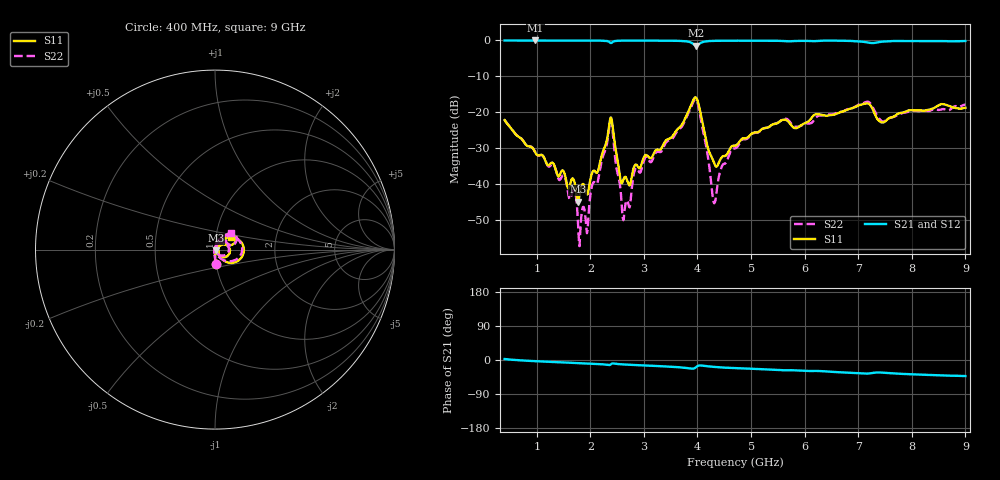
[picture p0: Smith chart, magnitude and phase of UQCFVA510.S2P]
!  Part Number  UQCFVA510  Mounting Orientation: Horizontal
!  Description: Ultra Low ESR Microwave capacitors
!  Application: Coupling, Bypass, Tuning, DC Block
!  Filters, Matching
# GHZ S DB R 50
! Freq  |S11|  S11 Ph  |S21|  S21 Ph  |S12|  S12 Ph  |S22|  S22 Ph
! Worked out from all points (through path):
!   801 points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, 400 MHz to 9 GHz, reference 50 ohm
!   highest |S21| = -0.02 dB at 970 MHz (marker M1); lowest = -1.5 dB at 3.98 GHz (marker M2)
!   group delay of S21, straight-line fit = 13.6 ps
!   lowest |S11| = -45.0 dB at 1.765 GHz (marker M3), VSWR 1.01, Z = 50.5 - j0.321 ohm
!   |S11| at or under -10 dB: start of sweep to end of sweep
!   |S22| runs from -57.3 to -16.4 dB; largest |S21 - S12| = 0.0062
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0.4  -22.20 -87.3  -0.04 2.5  -0.02 2.5  -22.15 -86.9
0.97  -31.17 -90.4  -0.02 -3.0  -0.01 -3.0  -31.10 -89.9
1.701  -39.32 -56.9  -0.03 -7.5  -0.01 -7.6  -41.82 -123.4
1.765  -44.95 -34.3  -0.03 -8.0  -0.01 -8.1  -49.64 -111.6
1.841  -40.37 -11.7  -0.03 -8.6  -0.02 -8.6  -47.86 160.7
1.948  -42.90 12.5  -0.04 -9.2  -0.02 -9.3  -52.94 115.1
2.034  -36.90 23.4  -0.04 -9.7  -0.03 -9.8  -40.33 97.0
2.152  -35.88 39.4  -0.06 -10.6  -0.05 -10.7  -38.32 79.9
2.378  -21.51 -1.2  -0.72 -12.0  -0.70 -12.1  -22.19 9.0
2.55  -37.56 -51.0  -0.09 -11.1  -0.07 -11.1  -40.05 -74.3
2.625  -38.49 -2.8  -0.06 -11.8  -0.05 -11.9  -49.45 55.2
2.84  -34.63 40.7  -0.06 -13.4  -0.05 -13.4  -35.77 82.1
3.27  -30.45 45.9  -0.07 -16.0  -0.05 -16.0  -31.03 79.9
3.98  -16.06 -12.2  -1.46 -18.2  -1.43 -18.3  -16.56 -8.8
4.313  -34.31 -13.6  -0.14 -18.2  -0.12 -18.4  -45.39 -1.9
4.442  -32.82 25.4  -0.10 -19.5  -0.08 -19.6  -35.61 64.0
4.7  -29.34 46.1  -0.09 -21.4  -0.06 -21.6  -30.12 73.3
5.603  -22.09 46.7  -0.18 -27.1  -0.17 -27.2  -21.92 53.5
6.141  -21.35 60.5  -0.21 -29.0  -0.20 -29.3  -22.85 61.9
7.162  -17.56 31.7  -0.54 -35.9  -0.53 -36.0  -17.10 31.8
7.57  -21.71 46.1  -0.22 -34.5  -0.19 -34.6  -21.72 40.6
9  -18.77 39.2  -0.18 -42.4  -0.17 -42.8  -17.88 46.0
